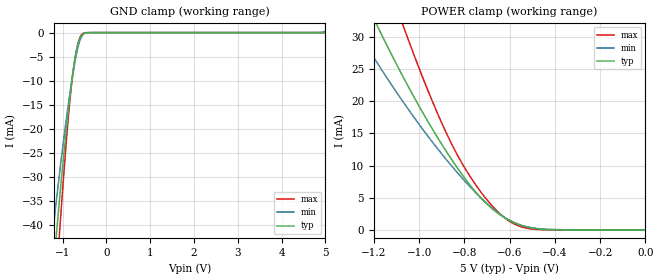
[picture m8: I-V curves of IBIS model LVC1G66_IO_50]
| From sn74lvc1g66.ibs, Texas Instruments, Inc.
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[Model]   LVC1G66_IO_50
Model_type  Terminator
| variable   typ   min   max
C_comp   5.49pF   3.77pF   6.04pF
| C_tri-state   5.49pF   3.77pF   6.04pF
[Temperature Range]   40   100   -40
| Ambient temperature   25   85   -40
[Voltage range]   5   4.5   5.5
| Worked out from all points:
|   GND clamp passes 1 mA (typ) near -0.59 V on its own axis
|   POWER clamp passes 1 mA (typ) near -0.57 V on its own axis
[GND Clamp]
| LVC1G66_IO_50
|   Voltage   I(typ)   I(min)   I(max)
-5.5V     -642.4mA   -532.1mA   -759.1mA
-1.235V   -51.96mA   -42.61mA   -64.15mA
-1.19V    -47.13mA   -38.88mA   -57.88mA
-1.145V   -42.4mA    -35.23mA   -51.73mA
-1.065V   -34.27mA   -28.96mA   -41.11mA
-895mV    -18.49mA   -16.7mA    -20.48mA
-785mV    -9.776mA   -9.773mA   -9.967mA
-715mV    -5.299mA   -5.981mA   -5.362mA
-655mV    -2.589mA   -3.308mA   -2.534mA
-590mV    -961uA     -1.29mA    -770.4uA
-515mV    -214.8uA   -272.3uA   -111.1uA
5V        244.7pA    324.5uA    53.99pA
[POWER Clamp]
| LVC1G66_IO_50
|   Voltage   I(typ)   I(min)   I(max)
-5.5V     606.3mA    485.7mA    811.7mA
-1.285V   39.21mA    31.62mA    54.52mA
-1.255V   36.91mA    29.88mA    51.12mA
-1.165V   30.26mA    24.84mA    41.31mA
-1.075V   24.05mA    20.1mA     32.16mA
-1.045V   22.08mA    18.59mA    29.27mA
-930mV    15.01mA    13.14mA    19.02mA
-825mV    9.336mA    8.655mA    11.26mA
-710mV    4.342mA    4.427mA    5.102mA
-620mV    1.861mA    1.909mA    1.83mA
-480mV    194.1uA    225.1uA    76.65uA
-95.1fV   244.7pA    1.173nA    65.01pA
